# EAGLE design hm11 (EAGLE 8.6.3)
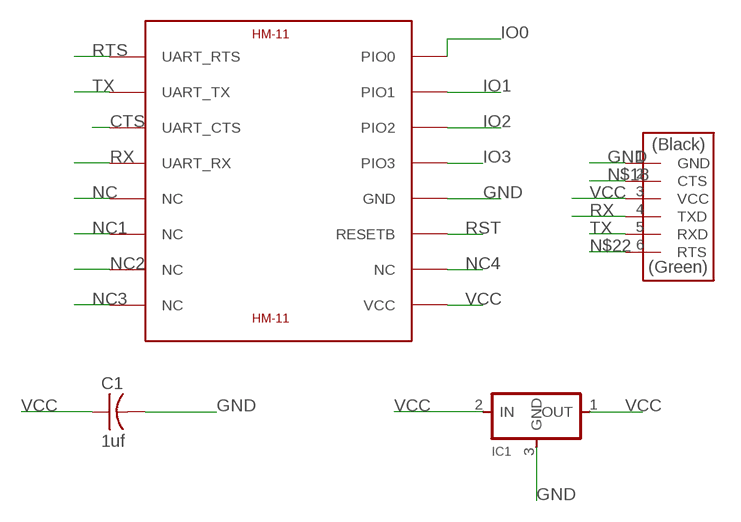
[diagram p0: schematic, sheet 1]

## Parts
C1  1uf  CAP-US1206FAB  [C1206FAB]
IC1  REGULATORSOT23  [SOT23]
U$1  HM-11  [HM-11]
U$2  FTDI-SMD-HEADER  [1X06SMD]

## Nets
CTS: U$1.UART_CTS
GND: C1.2 IC1.3(GND) U$1.GND U$2.1(GND)
IO0: U$1.PIO0
IO1: U$1.PIO1
IO2: U$1.PIO2
IO3: U$1.PIO3
N$18: U$2.2(CTS)
N$22: U$2.6(RTS)
NC: U$1.NC@5(NC)
NC1: U$1.NC@6(NC)
NC2: U$1.NC@7(NC)
NC3: U$1.NC@8(NC)
NC4: U$1.NC@10(NC)
RST: U$1.RESETB
RTS: U$1.UART_RTS
RX: U$1.UART_RX U$2.4(TXD)
TX: U$1.UART_TX U$2.5(RXD)
VCC: C1.1 IC1.1(OUT) IC1.2(IN) U$1.VCC U$2.3(VCC)

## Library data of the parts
C1 = fab:CAP-US
IC1 = fab:REGULATOR
U$1 = hm-11:HM-11: JNHuaMao HM-11 Bluetooth 4.0 Transceiver based on TI CC2540/CC2541
U$2 = fab:FTDI-SMD-HEADER

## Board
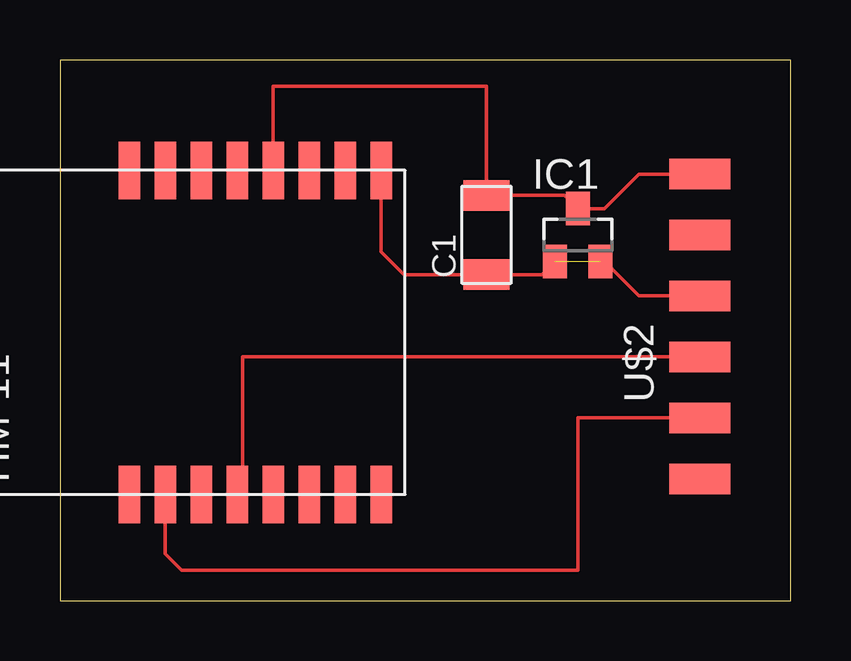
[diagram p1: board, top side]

Size 30.46 x 22.53 mm. Coordinates in mm from the lower left corner, seen from the top.
Outline: 0,0 30.46,0 30.46,22.53 0,22.53 0,0
Copper layers (1*16): Top 0.035mm / dielectric 1.5mm / Bottom 0.035mm
Design rules "default": minimum track width 6mil, minimum drill 0.35mm, track to track 6mil, track to pad 6mil, pad to pad 6mil, via to via 6mil, smd to smd 6mil, copper to edge 40mil, drill to drill 6mil, minimum pad ring 10mil, minimum via ring 8mil, stop-mask expansion 4mil, vias tented up to drill 0mil, thermal gap 10mil

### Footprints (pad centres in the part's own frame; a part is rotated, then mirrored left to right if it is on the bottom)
C1206FAB = smd 1.27 x 1.905: 1 -1.651,0; 2 1.651,0
SOT23 = smd 1 x 1.4: 1 -0.95,-1.1; 2 0.95,-1.1; 3 0,1.1
HM-11 = smd 2.4 x 0.9: GND 6.5,0; NC@5 -7,0; NC@6 -7,-1.5; NC@7 -7,-3; NC@8 -7,-4.5; NC@10 6.5,-3; PIO0 6.5,6; PIO1 6.5,4.5; PIO2 6.5,3; PIO3 6.5,1.5; RESETB 6.5,-1.5; UART_CTS -7,3; UART_RTS -7,6; UART_RX -7,1.5; UART_TX -7,4.5; VCC 6.5,-4.5
1X06SMD = smd 2.54 x 1.27: 1 0,6.35; 2 0,3.81; 3 0,1.27; 4 0,-1.27; 5 0,-3.81; 6 0,-6.35

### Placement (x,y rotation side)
C1  17.78,15.24 90 top
IC1  21.59,15.24 0 top
U$1  8.89,11.43 90 top
U$2  26.67,11.43 0 top

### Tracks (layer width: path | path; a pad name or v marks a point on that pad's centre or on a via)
GND
  Top 0.152: U$1.GND 8.89,21.44 17.78,21.44 C1.2 21.04,16.89 IC1.3 22.69,16.34 24.13,17.78 U$2.1
RX
  Top 0.152: U$1.UART_RX 7.62,4.66 7.62,10.16 U$2.4
TX
  Top 0.152: U$1.UART_TX 4.39,1.96 5.08,1.27 21.59,1.27 21.59,7.62 U$2.5
VCC  (1 unrouted)
  Top 0.152: U$1.VCC 13.39,14.55 14.35,13.59 C1.1 20.09,13.59 IC1.1 | IC1.2 22.69,14.14 24.13,12.7 U$2.3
